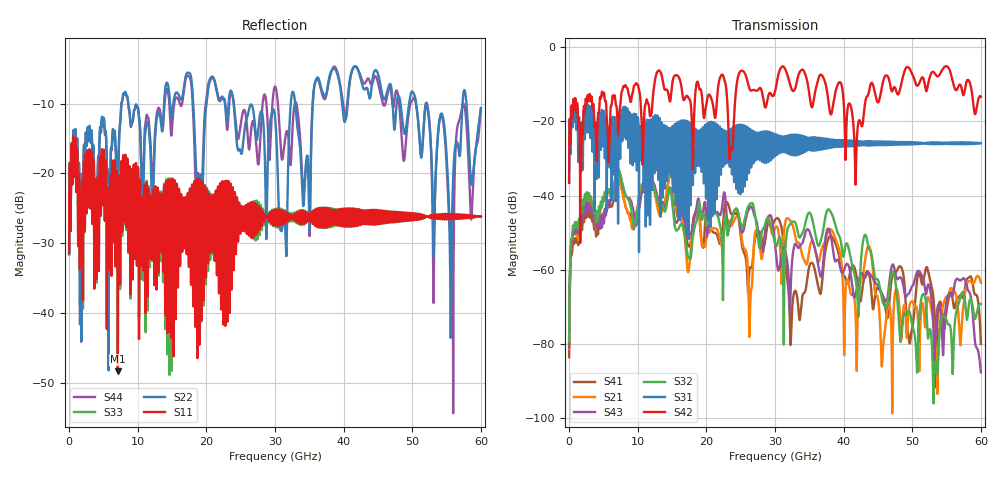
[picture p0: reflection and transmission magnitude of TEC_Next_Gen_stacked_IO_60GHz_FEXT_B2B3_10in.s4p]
!! CHANNEL DESCRIPTION:  Next Generation 28Gbps Press-fit Stacked I/O Connector
!!  with 10" 5-6-5 Megtron 6 Stripline trace on host side and 1.25" 7-5-7 Megtron 6 Microstrip trace on plug side
!! HOST PCB DESCRIPTION:  PCB thickness 3.425 mm
!!  26 Layer Board, 15 GND planes, 4 Layer route-out on Layers 7,11,17,21, 8mil stub on vias
!!  Pairs on following layers
!!  Layer 07 - A02A03 A14A15 D05D06
!!  Layer 11 - D020D3 C05C06 D14D15
!!  Layer 17 - C02C03 B05B06 C14C15
!!  Layer 21 - B02B03 A05A06 B14B15
!! CONNECTOR DESCRIPTION:  Next Generation 28Gbps Press-fit Stacked I/O Connector
!! PLUG-IN CARD DESCRIPTION:  PCB thickness 1mm thick
!!  6 Layer Board, 4 GND planes, 0.35 x 1.4mm mating pads
!!  Micro-strip diff traces referenced to GND plane 3mils down, 2nd GND plane 17mils from top of board
!!  PCB GND planes are symmetric
!! MODEL DESCRIPTION: TE Connectivity S-parameter model produced from Macro-model, Extracted .s4p FEXT (Victim B05B06 - Aggressor B02B03)
!! MODEL DATE: 5/15/2014 CR32f, FPR23
!! MODEL STATUS: Developmental
!! MODEL GEOMETRY: 4 Rows - Rows A, B, C, D. 3 pairs in each row, 12 total pairs
!! MODEL FREQUENCY RANGE: DC to 60 GHz in 10 MHz frequency steps
!! MODEL EDGE RATE LIMITATION: 8.33 ps (Using conservative 0.5/Fmax rule of thumb)
!! TIME-DOMAIN TRANSFORM CAUTIONS:
!! 1.) Do not simulate transient edge rates faster than the number listed above.  Edge
!!  rates faster than this number contain significant spectral content at frequencies
!!  above the model's highest frequency.
!! 2.) Even when simulating edge rates that are slower than the number listed above, be
!!  aware that the best time resolution possible with a direct iFFT is (1 / 2Fmax).
!!  As a result, time resolution is typically not adequate for most time-domain
!!  simulations unless tricks such as frequency-domain zero-padding and windowing are
!!  used to minimize leakage and aliasing.
!! 3.) Because the model has a uniform frequency step, a direct iFFT will result in an
!!  impulse that that has a time length given by either (1 / Fstep) or (1 / 2Fstep),
!!  depending on the transform being used.  Care has been taken in selecting the
!!  frequency step to ensure a settled impulse response for the model.  Therefore,
!!  convolution with the model's impulse response should present no issues.  However,
!!  if directly concatenating s-parameter models in the frequency domain a user must
!!  either interpolate necessary interim frequencies or complete impulse response
!!  zero-padding.  Impulse response zero-padding is more difficult, but more accurate.
!! PORT DEFINITIONS:
!! Port  1  ----->  Host B02		B05 Module <-----  Port  2
!! Port  3  ----->  Host B03		B06 Module <-----  Port  4
! Touchstone data
! Created: 29-Sep-2014 by IdEM R2011 (7.0.3)
# Hz S MA R 50
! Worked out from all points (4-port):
!   6000 points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, 10 MHz to 60 GHz, reference 50 ohm
!   strongest paths, dB at 10 MHz, 15.01 GHz, 30.01 GHz, 45.01 GHz, 60 GHz:
!     S42: -36.6, -10.1, -12.0, -14.9, -13.4
!     S31: -36.5, -24.6, -29.1, -25.6, -25.8
!     S32: -79.5, -41.6, -52.7, -62.8, -69.3
!     S43: -80.9, -40.6, -52.9, -64.3, -87.7
!     S21: -81.3, -35.7, -48.8, -68.0, -63.5
!     S41: -83.6, -34.9, -46.5, -64.9, -80.0
!   lowest |S11| = -48.4 dB at 7.11 GHz (marker M1), VSWR 1.01, Z = 50.2 + j0.308 ohm
!   |S11| at or under -10 dB: start of sweep to end of sweep
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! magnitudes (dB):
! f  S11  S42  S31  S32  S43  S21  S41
! 10 MHz  -31.4  -36.6  -36.5  -79.5  -80.9  -81.3  -83.6
! 7.11 GHz  -48.4  -22.9  -32.5  -33.3  -34.0  -35.6  -36.2
! 26.41 GHz  -24.4  -11.6  -22.7  -42.2  -43.0  -68.3  -59.3
! 43.68 GHz  -27.3  -12.2  -25.4  -54.3  -60.8  -53.7  -61.0
! 45.67 GHz  -25.8  -9.9  -25.9  -68.6  -66.9  -83.1  -66.9
! 55.58 GHz  -26.4  -6.9  -26.0  -75.8  -66.5  -65.0  -65.8
! 60 GHz  -26.2  -13.4  -25.8  -69.3  -87.7  -63.5  -80.0
